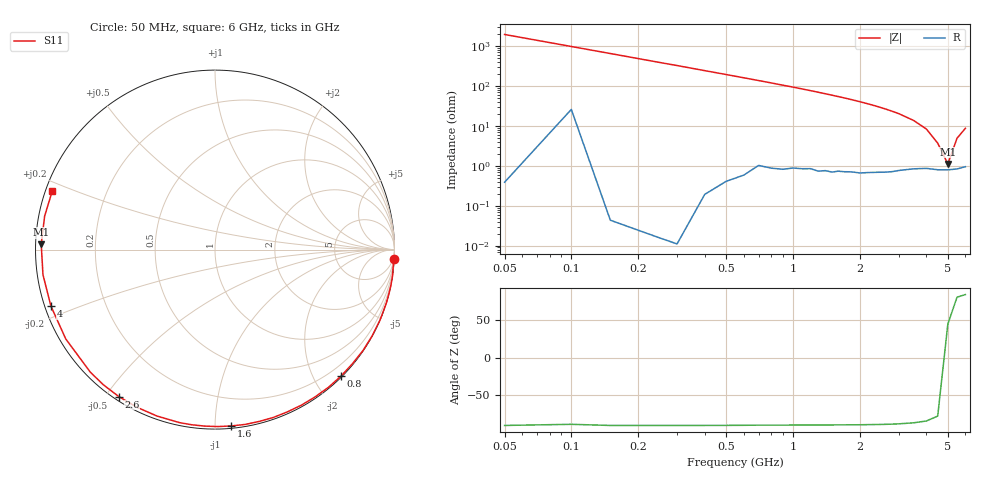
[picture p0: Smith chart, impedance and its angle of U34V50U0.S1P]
! SIEMENS Discrete & RF Semiconductors
! BBY53-02W
! Si Tuning Diode in SCD-80
! VR = 4.5 V
! S-Parameters:  September  1997
# GHz  S  MA  R  50
!  f  S11
! GHz  MAG  ANG
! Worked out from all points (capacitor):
!   34 points, 50 MHz to 6 GHz, reference 50 ohm
!   read as one part to ground: C = 1.61 pF near 50 MHz
!   lowest |Z| = 1.12 ohm at 5 GHz (marker M1)
!   series resonance near 4.911 GHz, so ESL is about 650 pH
!   S11 on the Smith chart (normalised r, x): 50 MHz: 0, -40; 800 MHz: 0.02, -2.40; 1.6 GHz: 0.01, -1.10; 2.6 GHz: 0.01, -0.54; 4 GHz: 0.02, -0.17; 6 GHz: 0.02, +0.17
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0.05  1 -2.9
0.2  1 -11.6
0.3  1 -17.3
0.4  0.9997 -23.1
0.5  0.999 -28.7
0.6  0.998 -34.3
0.8  0.9948 -45.2
0.9  0.994 -50.6
1  0.9923 -55.7
1.1  0.9913 -60.9
1.2  0.99 -65.9
1.3  0.9901 -70.8
1.4  0.9886 -75.6
1.5  0.9885 -80.2
1.6  0.9867 -84.7
1.8  0.985 -93.3
2  0.9842 -101.5
2.2  0.982 -109.2
2.4  0.9802 -116.4
2.6  0.9787 -123.2
2.8  0.9768 -129.6
3  0.974 -135.5
3.5  0.9691 -149.1
4  0.9668 -161.0
4.5  0.9686 -171.7
5  0.9686 178.2
5.5  0.9674 168.9
6  0.9636 160.2
